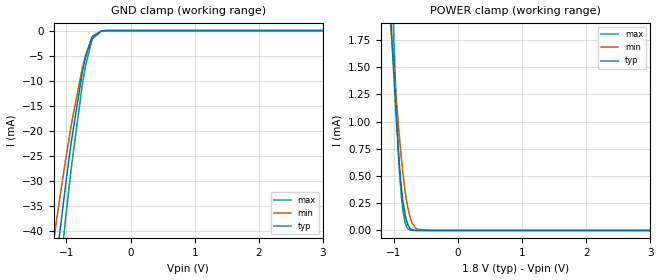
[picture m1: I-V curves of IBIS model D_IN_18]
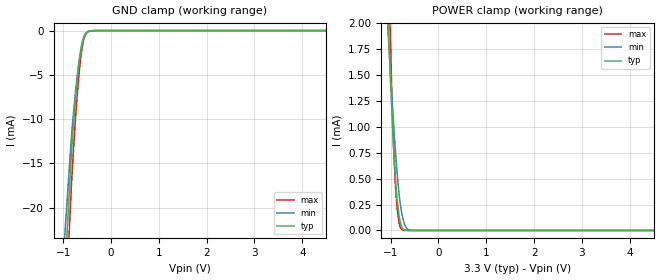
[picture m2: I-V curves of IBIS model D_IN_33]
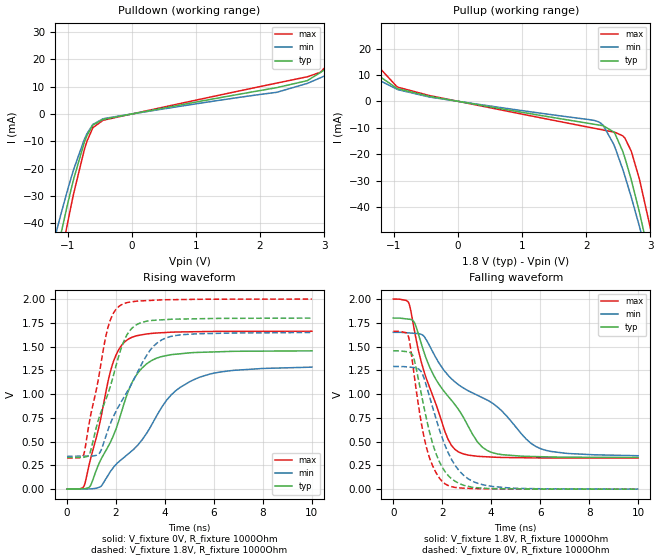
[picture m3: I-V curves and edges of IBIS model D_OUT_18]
| TEXAS INSTRUMENTS INCORPORATED
| Digital Video Dapartment/High Performance Analog
| IBIS Model of THS8200
| 'ALL-FORMAT' OVERSAMPLED COMPONENT VIDEO/PC GRAPHICS D/A SYSTEM
| This file contains package information for the following:
|  TQFP 80-pin (PFP) package as [Component] THS8200_PFP
| This device can be powered at the following Vccs:
|  1.8 volt, 3.3 volt Vcc
| This file provides unique models under the [Model Selector] for each Vcc.
| For operation at a specific Vcc, select the appropriate model after each
| [Model Selector] keyword.
[IBIS Ver]   4.1
[Comment char]  |_char
[File Name]   ths8200.ibs
[File Rev]   2.0
[Source]   Model built from spectre simulations at:
   Texas Instruments Incorporated.
   Analog-eLab, HPA
   12500 TI Blvd
   Dallas, TX -75243
   For Support e-mail: elab_ibis@list.ti.com
[Notes]   Revision History
   Rev 1.0: 02/09/2006.
   Rev 2.0: 03/04/2013. New, revised model with 1.8 and 3.3V buffers.
   - Pullup and Pulldown, non-monotonic on D_INOUT models.
   - Power Clamp on D_INOUT has odd dip, non-monotonic and result of circuit.
   - ccomp values are based on PVT settings:
   MIN: Low Voltage, High Temperature, Weak Process
   TYP: Nominal Voltage, Nominal Temperature, Nominal Process
   MAX: High Voltage, Low Temperature, Fast Process
   - C_comp although listed in numerical order of value are obtained from varying PVT conditions.
   For PVT conditions for each specific value, refer to the buffer description under respective [Model].
   IBIS model user is responsible for using appropriate C_comp to simulate for Signal Integrity.
[Disclaimer]  This model is designed as an aid for customers of Texas Instruments
 TI and its licensors and suppliers make no warranties, either expressed
 or implied, with respect to this  model, including the warranties of
 merchantability or fitness for a particular purpose.
 The model is provided solely on an "as is" basis. The entire risk as to
 its quality and performance is with the customer.
[Copyright] (C)Copyright 2013 Texas Instruments Incorporated.
   All rights reserved.
| Component THS8200_PFP 80-pin TQFP
[Component]   THS8200_PFP
[Manufacturer]   Texas Instruments, Inc.
[Package]
|   typ   min   max
R_pkg   4.000e-03   3.000e-03   4.000e-03
L_pkg   2.378e-09   2.123e-09   2.743e-09
C_pkg   4.750e-13   4.200e-13   5.340e-13
[Pin]   signal_name   model_name   R_pin   L_pin   C_pin
1   TESTMODE   D_IN   4.000e-03   2.743e-09   4.620e-13
2   GND_DLL   GND   4.000e-03   2.555e-09   5.340e-13
3   CLKIN   D_IN   4.000e-03   2.489e-09   5.230e-13
4   VDD_DLL   POWER   4.000e-03   2.431e-09   5.090e-13
5   IC2A   D_IN   4.000e-03   2.377e-09   4.960e-13
6   PBKG   GND   4.000e-03   2.328e-09   4.820e-13
7   FSADJ1   POWER   4.000e-03   2.286e-09   4.690e-13
8   FSADJ2   POWER   4.000e-03   2.250e-09   4.590e-13
9   COMP2   POWER   4.000e-03   2.222e-09   4.520e-13
10   COMP1   POWER   3.000e-03   2.127e-09   4.300e-13
11   AVDD   POWER   3.000e-03   2.127e-09   4.290e-13
12   AVSS   GND   4.000e-03   2.222e-09   4.520e-13
13   AGY   POWER   4.000e-03   2.250e-09   4.590e-13
14   AVDD   POWER   4.000e-03   2.285e-09   4.690e-13
15   ABPb   POWER   4.000e-03   2.329e-09   4.820e-13
16   AVSS   GND   4.000e-03   2.377e-09   4.960e-13
17   ARPr   POWER   4.000e-03   2.431e-09   5.100e-13
18   AVDD   POWER   4.000e-03   2.489e-09   5.230e-13
19   VDD_IO   POWER   4.000e-03   2.556e-09   5.340e-13
20   GND_IO   GND   4.000e-03   2.743e-09   4.620e-13
21   BCb9   D_IN   4.000e-03   2.660e-09   4.530e-13
22   BCb8   D_IN   4.000e-03   2.559e-09   5.290e-13
23   BCb7   D_IN   4.000e-03   2.493e-09   5.170e-13
24   BCb6   D_IN   4.000e-03   2.435e-09   5.030e-13
25   BCb5   D_IN   4.000e-03   2.381e-09   4.890e-13
26   BCb4   D_IN   4.000e-03   2.332e-09   4.750e-13
27   BCb3   D_IN   4.000e-03   2.289e-09   4.620e-13
28   BCb2   D_IN   4.000e-03   2.253e-09   4.520e-13
29   BCb1   D_IN   4.000e-03   2.225e-09   4.450e-13
30   BCb0   D_IN   3.000e-03   2.128e-09   4.240e-13
31   DVSS   GND   3.000e-03   2.127e-09   4.240e-13
32   DVDD   POWER   4.000e-03   2.225e-09   4.450e-13
33   RCr9   D_IN   4.000e-03   2.253e-09   4.520e-13
34   RCr8   D_IN   4.000e-03   2.289e-09   4.620e-13
35   RCr7   D_IN   4.000e-03   2.332e-09   4.750e-13
36   RCr6   D_IN   4.000e-03   2.381e-09   4.890e-13
37   RCr5   D_IN   4.000e-03   2.435e-09   5.030e-13
38   RCr4   D_IN   4.000e-03   2.493e-09   5.170e-13
39   RCr3   D_IN   4.000e-03   2.558e-09   5.290e-13
40   RCr2   D_IN   4.000e-03   2.649e-09   4.540e-13
41   RCr1   D_IN   4.000e-03   2.743e-09   4.580e-13
42   RCr0   D_IN   4.000e-03   2.557e-09   5.250e-13
43   HS_IN   D_INOUT   4.000e-03   2.492e-09   5.120e-13
44   VS_IN   D_INOUT   4.000e-03   2.434e-09   4.980e-13
45   GND_IO   GND   4.000e-03   2.380e-09   4.840e-13
46   VDD_IO   POWER   4.000e-03   2.331e-09   4.690e-13
47   FID   D_INOUT   4.000e-03   2.288e-09   4.570e-13
48   GY9   D_IN   4.000e-03   2.252e-09   4.460e-13
49   GY8   D_IN   4.000e-03   2.223e-09   4.400e-13
50   GY7   D_IN   3.000e-03   2.124e-09   4.200e-13
51   GY6   D_IN   3.000e-03   2.124e-09   4.200e-13
52   GY5   D_IN   4.000e-03   2.223e-09   4.400e-13
53   GY4   D_IN   4.000e-03   2.252e-09   4.460e-13
54   GY3   D_IN   4.000e-03   2.288e-09   4.570e-13
55   GY2   D_IN   4.000e-03   2.331e-09   4.690e-13
56   GY1   D_IN   4.000e-03   2.380e-09   4.840e-13
57   GY0   D_IN   4.000e-03   2.434e-09   4.980e-13
58   DVDD   POWER   4.000e-03   2.492e-09   5.120e-13
59   DVSS   GND   4.000e-03   2.557e-09   5.250e-13
60   REETB   D_IN   4.000e-03   2.743e-09   4.580e-13
61   HS_OUT   D_OUT   4.000e-03   2.656e-09   4.520e-13
62   VS_OUT   D_OUT   4.000e-03   2.556e-09   5.260e-13
63   SDA   D_INOUT   4.000e-03   2.490e-09   5.130e-13
64   SCL   D_INOUT   4.000e-03   2.433e-09   4.990e-13
65   DO9   D_OUT   4.000e-03   2.379e-09   4.840e-13
66   DO8   D_OUT   4.000e-03   2.330e-09   4.700e-13
67   DO7   D_OUT   4.000e-03   2.287e-09   4.570e-13
68   DO6   D_OUT   4.000e-03   2.251e-09   4.470e-13
69   DO5   D_OUT   4.000e-03   2.222e-09   4.410e-13
70   VDD_IO   POWER   3.000e-03   2.123e-09   4.200e-13
71   D1CLKO   D_OUT   3.000e-03   2.123e-09   4.200e-13
72   GND_IO   GND   4.000e-03   2.222e-09   4.410e-13
73   DO4   D_OUT   4.000e-03   2.250e-09   4.470e-13
74   DO3   D_OUT   4.000e-03   2.287e-09   4.570e-13
75   DO2   D_OUT   4.000e-03   2.330e-09   4.700e-13
76   DO1   D_OUT   4.000e-03   2.379e-09   4.840e-13
77   DO0   D_OUT   4.000e-03   2.433e-09   4.990e-13
78   DVSS   GND   4.000e-03   2.490e-09   5.130e-13
79   DVDD   POWER   4.000e-03   2.555e-09   5.260e-13
80   SCANEN   D_IN   4.000e-03   2.656e-09   4.520e-13
| Model D_IN
[Model Selector]   D_IN
D_IN_33   3.3 volt Vcc
D_IN_18   1.8 volt Vcc
| Model D_INOUT
[Model Selector]   D_INOUT
D_INOUT_33   3.3 volt Vcc
D_INOUT_18   1.8 volt Vcc
| Model D_OUT
[Model Selector]   D_OUT
D_OUT_33   3.3 volt Vcc
D_OUT_18   1.8 volt Vcc
| Models and submodels in the file (6): D_IN_18 (Input), D_IN_33 (Input), D_OUT_18 (Output), D_OUT_33 (Output), D_INOUT_33 (I/O_open_drain), D_INOUT_18 (I/O_open_drain)
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[Model]   D_IN_18
Model_type   Input
Vinl = .4
Vinh = 0.95
|   typ   min   max
C_comp   1.273p   1.273p   1.273p
[Voltage Range]   1.8   1.65   2
[Temperature Range]   27   85   0
[Power Clamp Reference]   1.8   1.65   2
[GND Clamp Reference]   -0   -0   -0
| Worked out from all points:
|   GND clamp passes 1 mA (typ) near -0.57 V on its own axis
|   POWER clamp passes 1 mA (typ) near -0.96 V on its own axis
[GND Clamp]
|   Voltage   I(typ)   I(min)   I(max)
-1.8V     -147.6mA   -110mA     -175.3mA
-1.206V   -51.49mA   -42.55mA   -61.5mA
-1.147V   -44.91mA   -37.2mA    -53.9mA
-1.136V   -43.73mA   -36.24mA   -52.54mA
-1.012V   -30.73mA   -25.7mA    -37.42mA
-919.8mV  -21.9mA    -18.54mA   -27.05mA
-752.4mV  -8.409mA   -7.53mA    -10.9mA
-703.8mV  -5.446mA   -5.069mA   -7.232mA
-606.6mV  -1.498mA   -1.635mA   -2.103mA
-590.4mV  -1.123mA   -1.279mA   -1.587mA
-450mV    -40.25uA   -77.17uA   -52.05uA
3.595V    0A         0A         0A
[POWER Clamp]
|   Voltage   I(typ)   I(min)   I(max)
-1.8V     11.58mA    8.478mA    19.36mA
-1.039V   1.848mA    1.8mA      2.468mA
-1.006V   1.488mA    1.544mA    1.87mA
-941.4mV  837.3uA    1.057mA    863.7uA
-892.8mV  456.9uA    727.4uA    383.5uA
-860.4mV  279uA      535.6uA    194.6uA
-822.6mV  140.9uA    351.7uA    69.7uA
-774mV    43.68uA    185.9uA    12.82uA
-709.2mV  5.428uA    61.15uA    1.034uA
-644.4mV  539.3nA    12.64uA    73.51nA
-450mV    0A         32.76nA    0A
3.595V    0A         0A         0A
[Model]   D_IN_33
Model_type   Input
Vinl = 1.15
Vinh = 2.3
|   typ   min   max
C_comp   1.273p   1.273p   1.273p
[Voltage Range]   3.3   3   3.6
[Temperature Range]   27   85   0
[Power Clamp Reference]   3.3   3   3.6
[GND Clamp Reference]   -0   -0   -0
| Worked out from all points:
|   GND clamp passes 1 mA (typ) near -0.58 V on its own axis
|   POWER clamp passes 1 mA (typ) near -0.96 V on its own axis
[GND Clamp]
|   Voltage   I(typ)   I(min)   I(max)
-3.3V     -1.546A    -1.457A    -1.589A
-1.181V   -48.74mA   -40.31mA   -58.33mA
-825mV    -13.74mA   -11.9mA    -17.35mA
-775.5mV  -10mA      -8.841mA   -12.84mA
-726mV    -6.73mA    -6.14mA    -8.833mA
-686.4mV  -4.532mA   -4.298mA   -6.077mA
-646.8mV  -2.778mA   -2.789mA   -3.815mA
-607.2mV  -1.513mA   -1.65mA    -2.124mA
-567.6mV  -720.6uA   -877.8uA   -1.023mA
-528mV    -301.3uA   -420.2uA   -424.2uA
-478.5mV  -87.36uA   -147.8uA   -117.7uA
6.59V     0A         0A         0A
[POWER Clamp]
|   Voltage   I(typ)   I(min)   I(max)
-3.3V     31.72mA    22.25mA    54.41mA
-1.073V   2.239mA    2.075mA    3.13mA
-1.023V   1.673mA    1.676mA    2.175mA
-1.013V   1.563mA    1.598mA    1.994mA
-933.9mV  770.9uA    1.003mA    772uA
-894.3mV  466.7uA    736.9uA    394.4uA
-864.6mV  298.6uA    558.8uA    214.4uA
-825mV    147.8uA    361.9uA    75.04uA
-745.8mV  18.59uA    120.4uA    4.346uA
-666.6mV  1.196uA    22.76uA    181.3nA
-528mV    0A         405.9nA    0A
6.59V     0A         0A         0A
[Model]   D_OUT_18
Model_type   Output
Polarity   Non-Inverting
Vmeas = 0.9
Vref = 0.9
Cref = 15pF
Rref = 1000
|   typ   min   max
C_comp   1.273p   1.273p   1.273p
[Voltage Range]   1.8   1.65   2
[Temperature Range]   27   85   0
[Pullup Reference]   1.8   1.65   2
[Pulldown Reference]   -0   -0   -0
[Power Clamp Reference]   1.8   1.65   2
[GND Clamp Reference]   -0   -0   -0
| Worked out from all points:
|   slope of the pulldown table from 0 to 0.27 V, typ, clamps not added: 227 ohm
|   slope of the pullup table from 0 to 0.27 V, typ, clamps not added: 237 ohm
|   falling waveform, V_fixture 1.8V, R_fixture 1000Ohm: 20-80 % time 1.96ns typ, 3.41ns min, 1.17ns max; typ from 1.8 V to 0.333 V
|   rising waveform, V_fixture 0V, R_fixture 1000Ohm: 20-80 % time 1.4ns typ, 2.41ns min, 904ps max; typ from 0 V to 1.46 V
|   rising waveform, V_fixture 1.8V, R_fixture 1000Ohm: 20-80 % time 1.07ns typ, 1.55ns min, 755ps max; typ from 0.332 V to 1.8 V
|   falling waveform, V_fixture 0V, R_fixture 1000Ohm: 20-80 % time 858ps typ, 1.09ns min, 691ps max; typ from 1.46 V to 0 V
[Pulldown]
|   Voltage   I(typ)   I(min)   I(max)
-1.8V     -150.2mA   -113.5mA   -177.7mA
-1.163V   -50.38mA   -41.95mA   -60.08mA
-1.109V   -44.41mA   -37.09mA   -53.18mA
-1.006V   -33.58mA   -28.27mA   -40.58mA
-903.6mV  -23.62mA   -20.15mA   -28.89mA
-698.4mV  -7.925mA   -7.219mA   -9.996mA
-606.6mV  -4.051mA   -3.824mA   -5.013mA
-450mV    -2.02mA    -1.777mA   -2.338mA
2.261V    9.641mA    7.938mA    11.31mA
2.736V    12.2mA     11.19mA    13.61mA
2.941V    15.18mA    13.25mA    15.27mA
3.595V    25.69mA    19.94mA    31.8mA
[Pullup]
|   Voltage   I(typ)   I(min)   I(max)
-1.8V     19.11mA    15.01mA    27.92mA
-936mV    4.728mA    4.412mA    5.332mA
-450mV    1.907mA    1.636mA    2.205mA
2.191V    -8.961mA   -7.794mA   -10.53mA
2.266V    -9.296mA   -9.185mA   -10.89mA
2.45V     -12.39mA   -17.63mA   -11.78mA
2.569V    -18.98mA   -25.8mA    -13.07mA
2.601V    -21.35mA   -28.26mA   -13.92mA
2.704V    -29.95mA   -36.53mA   -19.1mA
2.828V    -41.97mA   -47.34mA   -29.47mA
3.011V    -61.86mA   -64.46mA   -49.36mA
3.595V    -150.6mA   -190.7mA   -127.1mA
[Ramp]
R_load = 1000
|   typ   min   max
dV/dt_r   0.873061/1.3982e-09   0.770207/2.4119e-09   0.996785/9.04351e-10
dV/dt_f   0.88028/1.96227e-09   0.778958/3.41458e-09   1.00369/1.17239e-09
[Falling Waveform]
V_fixture = 1.8V
V_fixture_min = 1.65V
V_fixture_max = 2V
R_fixture = 1000Ohm
C_fixture = 0F
|   Time   V(typ)   V(min)   V(max)
0s        1.8V       1.65V      2V
636.8ps   1.788V     1.644V     1.957V
866.1ps   1.751V     1.64V      1.666V
1.274ns   1.427V     1.602V     1.223V
2.23ns    980.1mV    1.201V     528.1mV
2.662ns   838.9mV    1.099V     391.9mV
3.442ns   495.9mV    987.1mV    345.7mV
4.042ns   384.2mV    906mV      337.6mV
6.021ns   341.6mV    425.3mV    328.5mV
10ns      332.9mV    351.7mV    327.2mV
[Rising Waveform]
V_fixture = 0V
V_fixture_min = 0V
V_fixture_max = 0V
R_fixture = 1000Ohm
C_fixture = 0F
|   Time   V(typ)   V(min)   V(max)
0s        1.018nV    6.879nV    812.8pV
700.4ps   4.389mV    2.137mV    35.52mV
953.2ps   35.35mV    2.908mV    310.7mV
1.365ns   301.4mV    25.6mV     727.2mV
1.837ns   530.6mV    208.4mV    1.298V
2.518ns   1.042V     375.1mV    1.581V
3.442ns   1.352V     670.6mV    1.638V
4.246ns   1.415V     989.4mV    1.651V
5.221ns   1.438V     1.157V     1.656V
10ns      1.455V     1.284V     1.661V
[Rising Waveform]
V_fixture = 1.8V
V_fixture_min = 1.65V
V_fixture_max = 2V
R_fixture = 1000Ohm
C_fixture = 0F
|   Time   V(typ)   V(min)   V(max)
0s        332.4mV    345.2mV    327.2mV
683ps     335mV      347.5mV    365.5mV
929.1ps   375.3mV    348.4mV    730mV
1.326ns   766.1mV    379.2mV    1.228V
1.676ns   1.008V     625.1mV    1.706V
2.23ns    1.495V     925.9mV    1.941V
2.763ns   1.718V     1.17V      1.975V
3.407ns   1.773V     1.467V     1.986V
4.07ns    1.785V     1.594V     1.993V
10ns      1.8V       1.648V     2V
[Falling Waveform]
|Gnd
V_fixture = 0V
V_fixture_min = 0V
V_fixture_max = 0V
R_fixture = 1000Ohm
C_fixture = 0F
|   Time   V(typ)   V(min)   V(max)
0s        1.456V     1.291V     1.661V
596.6ps   1.445V     1.286V     1.622V
828.6ps   1.386V     1.28V      1.249V
1.142ns   1.007V     1.235V     701.6mV
1.354ns   741.7mV    1.085V     438.8mV
1.663ns   434.4mV    811.8mV    215.6mV
2.114ns   184.8mV    460.8mV    56.21mV
2.709ns   58.08mV    187.5mV    13.32mV
3.719ns   9.762mV    42.99mV    4.486mV
10ns      59.59uV    447.8uV    5.394uV
